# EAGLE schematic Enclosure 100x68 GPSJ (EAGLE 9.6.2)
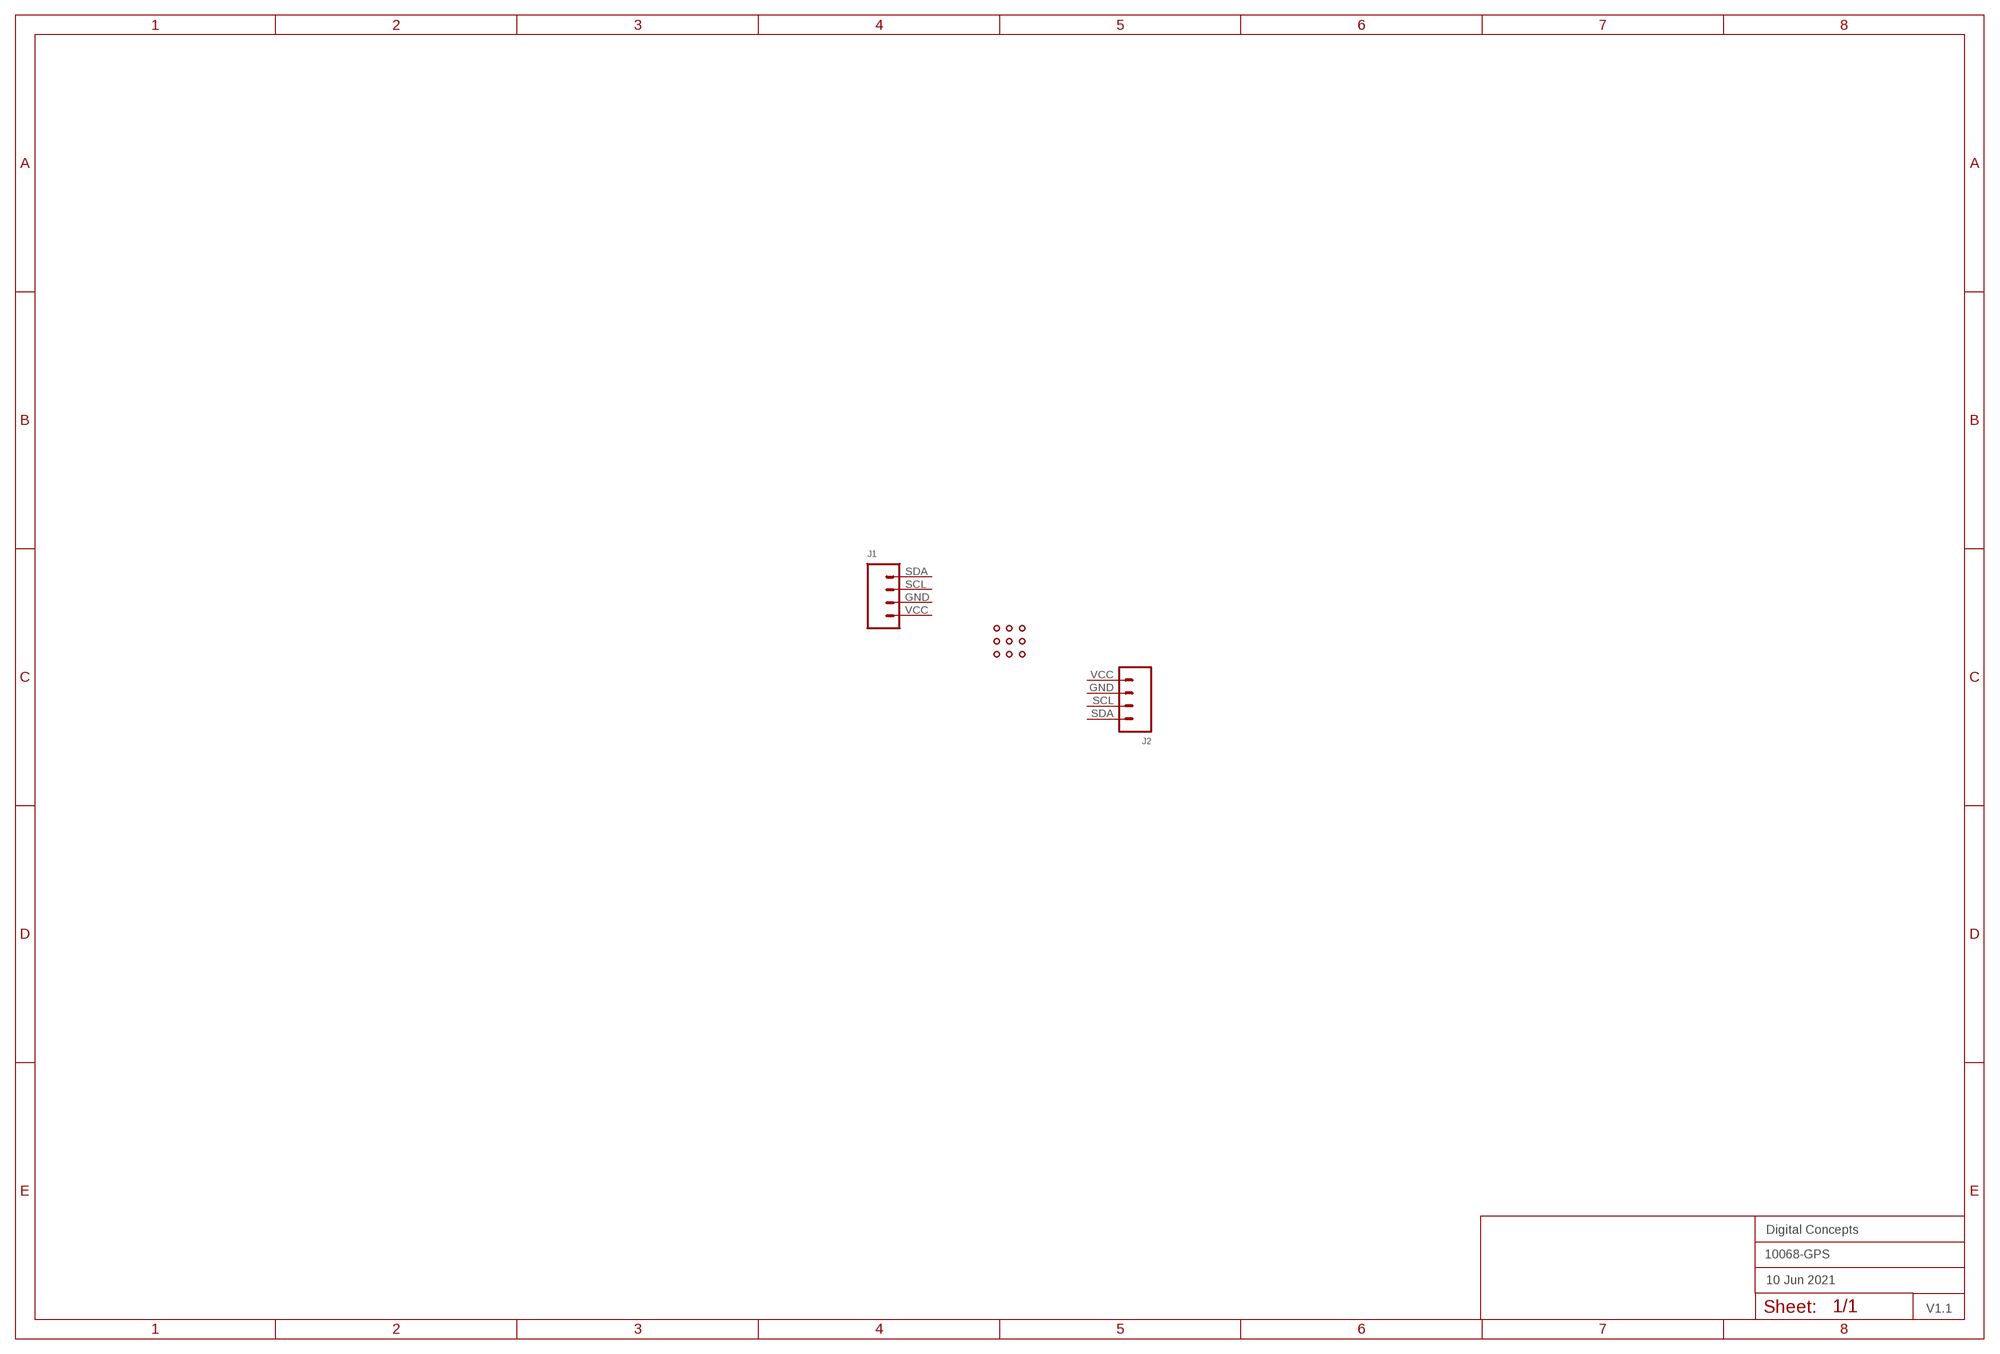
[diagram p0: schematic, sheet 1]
FRAME2 (A3L-LOC): DATE: 10 Jun 2021; OWNER: Digital Concepts; TITLE: 10068-GPS; VERSION: V1.1

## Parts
J1  JST-PH2.0-I2C-MALE-HORIZONTAL  [JST-PH2.0-4-HORIZONTAL]
J2  JST-PH2.0-I2C-MALE-HORIZONTAL  [JST-PH2.0-4-HORIZONTAL]
U$1  PROTO-34X22-GPS-I2C  [PROTO-34X22-GPS-I2C]
Unconnected: J1.GND J1.SCL J1.SDA J1.VCC J2.GND J2.SCL J2.SDA J2.VCC

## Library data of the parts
J1 J2 = digitalconcepts:JST-PH2.0-I2C-MALE-HORIZONTAL: PH2.0 4P (I2C) Right Angle PCB Connector
U$1 = digitalconcepts:PROTO-34X22-GPS-I2C: 34 x 22 Prototyping board to fit an 100 x 68 enclosure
